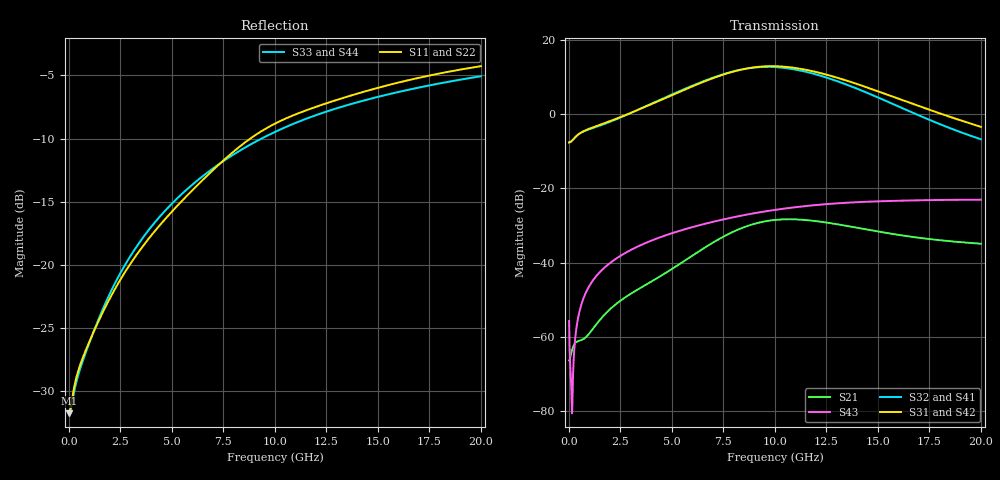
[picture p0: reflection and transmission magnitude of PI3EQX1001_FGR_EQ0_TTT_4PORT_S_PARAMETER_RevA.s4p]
! NPort=4 DATA=2000 NOISE=0 GROUPDELAY=0 COMPLEX_DATAFORMAT=POLAR
! NumOfBlock=1 NumOfParam=0
! .MODEL Smodel S TSTONEFILE=PI3EQX1001_FGR_EQ0_TTT_4PORT_S_PARAMETER_RevA.s4p TYPE=S
!  -- The above .MODEL line can be used for the S element in the netlist.
! The s parameter is extracted from the linear redriver, it is not bi-directional; only s(4,1)s(4,2) and s(3,1)s(3,2)
! should be the insertion loss
!Port definition:
!Port1 = input+
!Port2 = input¨C
!Port3 = output+
!Port4 = output-
# Hz S MA R  50
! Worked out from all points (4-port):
!   2000 points, 10 MHz to 20 GHz, reference 50 ohm
!   strongest paths, dB at 10 MHz, 5.01 GHz, 10.01 GHz, 15.01 GHz, 20 GHz:
!     S31: -7.6, 5.2, 13.0, 6.2, -3.4
!     S42: -7.6, 5.2, 12.9, 6.2, -3.4
!     S32: -7.6, 5.4, 12.7, 4.5, -6.7
!     S41: -7.6, 5.3, 12.7, 4.5, -6.8
!     S43: -55.8, -32.1, -25.8, -23.5, -23.1
!     S21: -66.4, -41.7, -28.5, -31.6, -34.9
!   lowest |S11| = -31.7 dB at 10 MHz (marker M1), VSWR 1.05, Z = 47.5 - j0.063 ohm
!   |S11| at or under -10 dB: start of sweep to 8.811 GHz
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1e7  0.0259 -178.5  0.0004911 2.7  3.669e-05 -0.2  4.787e-05 -0.1
     0.0004778 2.9  0.02597 -178.7  4.577e-05 -0.2  5.994e-05 -0.1
     0.417 0.1  0.417 -179.9  0.02616 178.4  0.001615 -59.2
     0.4168 -179.9  0.4169 0.1  0.001626 -59.0  0.02612 178.4
6.66e9  0.2234 -104.9  0.01565 94.6  2.235e-05 -30.9  3.237e-05 -29.5
        0.01632 92.8  0.2217 -104.8  2.946e-05 -26.2  4.098e-05 -24.7
        2.827 -52.0  2.879 132.0  0.2298 -111.4  0.03362 58.8
        2.868 131.9  2.82 -52.0  0.03362 58.8  0.2298 -111.4
8.77e9  0.3145 -107.7  0.03077 63.1  1.999e-05 -28.0  3.206e-05 -31.8
        0.03181 61.7  0.3124 -107.7  2.991e-05 -25.7  3.87e-05 -24.6
        4.208 -111.2  4.188 72.9  0.2981 -114.1  0.04513 46.2
        4.167 73.0  4.2 -111.1  0.04506 46.1  0.298 -114.0
1.069e10  0.3844 -113.4  0.03714 26.1  2.191e-05 -22.4  3.364e-05 -41.6
          0.03835 24.9  0.3815 -113.5  3.196e-05 -34.8  4.019e-05 -23.8
          4.313 -173.0  4.14 11.6  0.3556 -117.3  0.05463 33.3
          4.116 11.8  4.306 -172.9  0.05445 33.2  0.3554 -117.2
1.32e10  0.4546 -118.9  0.03116 -8.6  2.889e-05 -37.3  3.053e-05 -64.2
         0.03222 -9.6  0.4508 -119.0  2.878e-05 -55.6  4.61e-05 -34.7
         3.009 115.4  2.685 -58.6  0.4211 -121.6  0.06351 16.0
         2.667 -58.4  3.004 115.5  0.06335 16.1  0.421 -121.5
1.573e10  0.5198 -123.5  0.02337 -24.9  2.867e-05 -69.7  2.233e-05 -93.6
          0.02427 -26.0  0.5154 -123.6  2.009e-05 -81.5  4.322e-05 -57.1
          1.722 58.9  1.375 -111.3  0.4774 -125.4  0.06795 0.1
          1.365 -110.8  1.719 59.0  0.06787 0.2  0.4771 -125.4
2e10  0.611 -130.8  0.0173 -32.9  1.522e-05 -148.6  1.288e-05 149.9
      0.01794 -34.8  0.6056 -130.9  8.704e-06 135.5  1.803e-05 -97.0
      0.6765 -9.5  0.4599 -161.9  0.5574 -131.1  0.0704 -23.6
      0.4579 -161.0  0.6745 -9.3  0.07036 -23.6  0.5573 -131.1
